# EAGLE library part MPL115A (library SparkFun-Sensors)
NXP MPL115A 50 to 115kPa, Absolute Digital Pressure Sensor The MPL115A is a simple barometer with digital output for cost-effective applications. It employs a MEMS pressure sensor with a conditioning integrated circuit to provide accurate pressure data. An integrated analog-to-digital converter (ADC) provides digitized temperature and pressure sensor outputs via either a serial peripheral interface (SPI) (MPL115A1) or I²C (MPL115A2) port. Datasheet SparkFun Products SparkFun Barometric Pressure Sensor Breakout - MPL115A1 (SEN-09721) Barometric Pressure Sensor - MPL115A1 (SEN-09602)
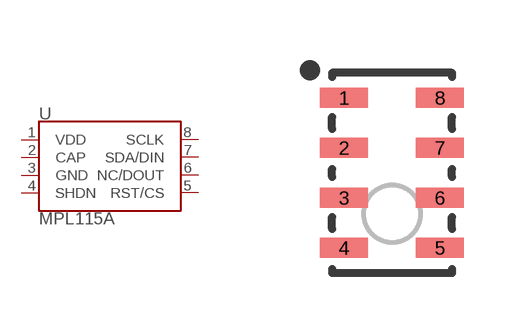
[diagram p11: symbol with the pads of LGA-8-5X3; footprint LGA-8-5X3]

Designator prefix U

## MPL115A (PROD_ID: IC-09492; SF_ID: SEN-09602)  [LGA-8-5X3]
1  VDD
2  CAP
3  GND
4  SHDN
5  RST/CS
6  NC/DOUT
7  SDA/DIN
8  SCLK

## Footprint LGA-8-5X3 (pad centres in mm)
8-Pin Land Grid Array (LGA) (5 x 3 mm) Datasheet Specifications: Pin Count: 8 Area: 5.0 x 3.0 x 1.2 mm Pitch: 1.25 mm Devices Using: MPL115A MPL3115A2
smd 1.2 x 0.5: 1 -1.2,1.875; 2 -1.2,0.625; 3 -1.2,-0.625; 4 -1.2,-1.875; 5 1.2,-1.875; 6 1.2,-0.625; 7 1.2,0.625; 8 1.2,1.875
